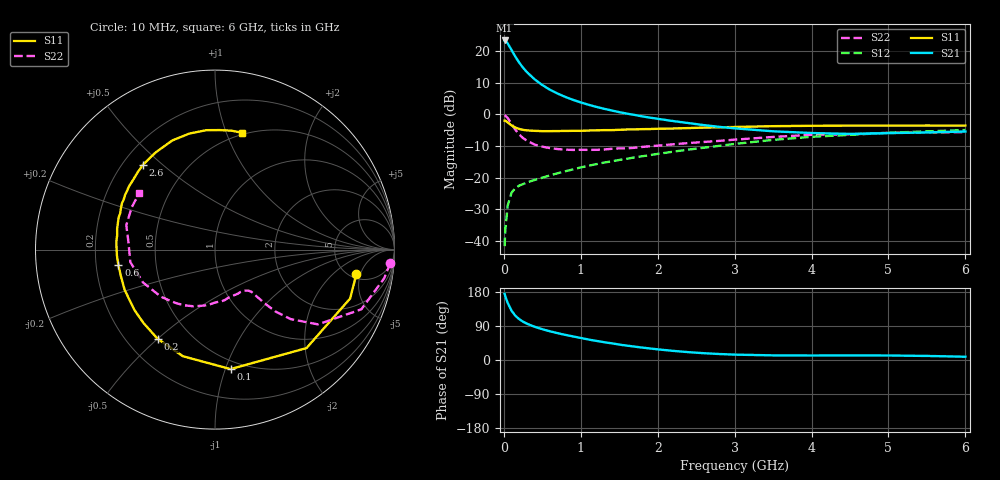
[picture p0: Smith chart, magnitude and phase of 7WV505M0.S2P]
! Infineon Technologies  Discrete & RF Semiconductors
! BFS17W
! Si NPN RF Bipolar Junction Transistor in SOT323
! VCE = 0.5 V  IC = 5 mA
! Common Emitter S-Parameters:  August  1999
# GHz  S  MA  R  50
!  f  S11  S21  S12  S22
! GHz  MAG  ANG  MAG  ANG  MAG  ANG  MAG  ANG
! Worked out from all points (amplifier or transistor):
!   36 points, 10 MHz to 6 GHz, reference 50 ohm
!   highest |S21| = 23.4 dB at 10 MHz (marker M1)
!   |S21| within 3 dB of that: start of sweep to 99.83 MHz
!   unconditionally stable (mu >= 1): 446.8 MHz to end of sweep
!   at 250 MHz: K = 0.67, MSG = 18.4 dB, |S12| = -22.0 dB
!   at 1.4 GHz: K = 1.43, MAG = 4.1 dB, |S12| = -14.8 dB
!   at 6 GHz: K = 1.15, MAG = -2.6 dB, |S12| = -4.9 dB
!   S11 on the Smith chart (normalised r, x): 10 MHz: 5.64, -4.29; 100 MHz: 0.43, -1.04; 200 MHz: 0.33, -0.50; 600 MHz: 0.30, -0.07; 2.6 GHz: 0.28, +0.43; 6 GHz: 0.48, +1.13
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0.01  0.7995 -9.9  14.77 174.4  0.0083 80.7  0.9799 -4.4
0.02  0.8007 -19.9  14.68 167.6  0.0155 80.0  0.9562 -9.6
0.05  0.749 -47.1  13.26 150.6  0.0363 67.2  0.8806 -22.2
0.1  0.6714 -82.6  10.45 130.2  0.0581 52.2  0.7089 -36.0
0.15  0.6203 -106.8  8.167 116.7  0.0687 44.2  0.5718 -42.6
0.2  0.5909 -122.8  6.601 107.7  0.0753 41.3  0.4845 -45.6
0.25  0.5707 -134.4  5.472 101.1  0.0794 39.3  0.4226 -46.9
0.3  0.5608 -143.4  4.662 95.9  0.0843 39.5  0.3852 -47.6
0.4  0.5512 -156.0  3.592 87.7  0.0923 40.5  0.3344 -48.7
0.5  0.5448 -164.5  2.918 81.3  0.1002 42.5  0.3101 -49.2
0.6  0.5451 -171.0  2.456 75.7  0.109 44.2  0.2943 -50.9
0.7  0.5473 -176.3  2.136 70.8  0.1179 45.5  0.284 -53.6
0.8  0.5488 179.0  1.892 66.2  0.1267 46.8  0.2782 -56.6
1.1  0.5577 167.9  1.424 54.1  0.1546 49.1  0.2756 -66.9
1.3  0.5659 161.5  1.232 47.1  0.1734 49.6  0.2793 -75.3
1.6  0.579 153.6  1.031 37.9  0.1997 50.1  0.2922 -87.3
2.2  0.5997 139.3  0.787 24.1  0.2582 49.7  0.3377 -110.7
2.6  0.62 130.4  0.679 17.9  0.2982 48.2  0.3678 -125.5
3.5  0.653 111.4  0.542 12.2  0.3965 41.5  0.4412 -155.5
4.5  0.6671 94.1  0.493 12.1  0.4759 30.6  0.4847 174.7
5.5  0.6691 81.9  0.52 10.7  0.5404 21.0  0.5204 153.0
6  0.6679 77.2  0.538 8.6  0.5678 16.3  0.5265 143.3
